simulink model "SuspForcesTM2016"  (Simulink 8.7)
settings: Solver=VariableStepAuto  SolverMode=SingleTasking  StartTime=0.0  StopTime=10.0  RelTol=1e-3

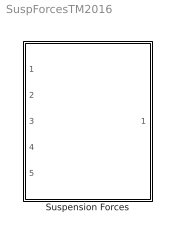
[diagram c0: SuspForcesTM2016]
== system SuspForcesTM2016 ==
  Suspension Forces : Subsystem

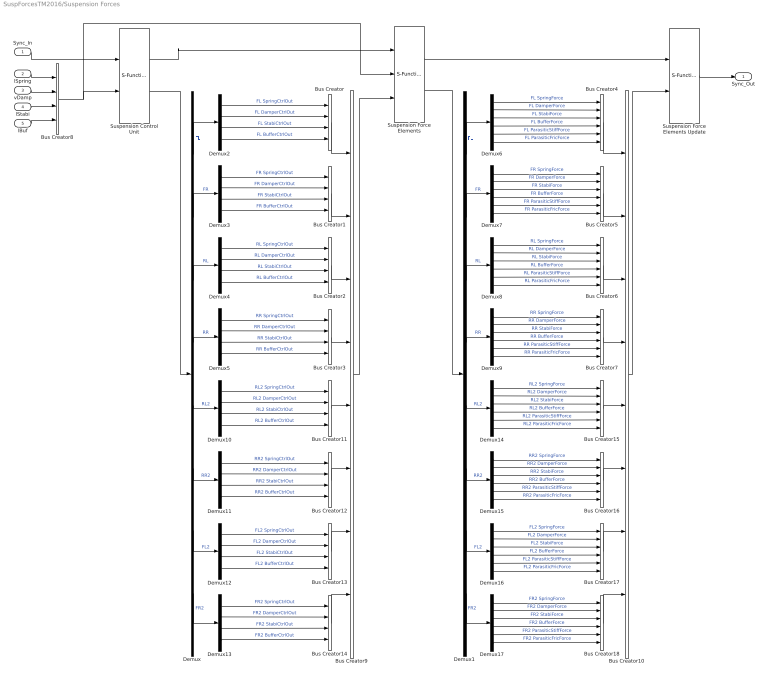
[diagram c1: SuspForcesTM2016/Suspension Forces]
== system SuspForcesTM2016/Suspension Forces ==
  Sync_In : Inport
  lSpring : Inport  Port=2
  vDamp : Inport  Port=3
  lStabi : Inport  Port=4
  lBuf : Inport  Port=5
  Bus Creator{,1..3,8,11..14} (9 alike) : BusCreator  Inputs=4
  Bus Creator10 : BusCreator  Inputs=8
  Bus Creator{4..7,15..18} (8 alike) : BusCreator  Inputs=6
  Bus Creator9 : BusCreator  Inputs=8
  Demux : Demux  Outputs=8
  Demux1 : Demux  Outputs=8
  Demux{2..5,10..13} (8 alike) : Demux
  Demux{6..9,14..17} (8 alike) : Demux  Outputs=6
  Suspension Control Unit : S-Function  FunctionName=TM_Sfun  Parameters='ForcesSuspControl'  SFunctionDeploymentMode=off  EnableBusSupport=off
  Suspension Force Elements : S-Function  FunctionName=TM_Sfun  Parameters='ForcesSusp'  SFunctionDeploymentMode=off  EnableBusSupport=off
  Suspension Force Elements Update : S-Function  FunctionName=TM_Sfun  Parameters='ForcesSuspUpd'  SFunctionDeploymentMode=off  EnableBusSupport=off
  Sync_Out : Outport
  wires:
  vDamp/1 -> Bus Creator8/2
  lStabi/1 -> Bus Creator8/3
  lBuf/1 -> Bus Creator8/4
  lSpring/1 -> Bus Creator8/1
  Bus Creator8/1 -> Suspension Control Unit/2, Suspension Force Elements/2
  Sync_In/1 -> Suspension Control Unit/1
  Suspension Control Unit/1 -> Suspension Force Elements/1
  Suspension Force Elements/1 -> Suspension Force Elements Update/1
  Suspension Force Elements Update/1 -> Sync_Out/1
  Bus Creator4/1 -> Bus Creator10/1
  Bus Creator5/1 -> Bus Creator10/2
  Bus Creator6/1 -> Bus Creator10/3
  Bus Creator7/1 -> Bus Creator10/4
  Demux6/1 -> Bus Creator4/1  "FL SpringForce"
  Demux9/1 -> Bus Creator7/1  "RR SpringForce"
  Demux9/2 -> Bus Creator7/2  "RR DamperForce"
  Demux9/3 -> Bus Creator7/3  "RR StabiForce"
  Demux9/4 -> Bus Creator7/4  "RR BufferForce"
  Demux9/5 -> Bus Creator7/5  "RR ParasiticStiffForce"
  Demux9/6 -> Bus Creator7/6  "RR ParasiticFricForce"
  Demux8/1 -> Bus Creator6/1  "RL SpringForce"
  Demux8/2 -> Bus Creator6/2  "RL DamperForce"
  Demux8/4 -> Bus Creator6/4  "RL BufferForce"
  Demux8/5 -> Bus Creator6/5  "RL ParasiticStiffForce"
  Demux8/6 -> Bus Creator6/6  "RL ParasiticFricForce"
  Demux8/3 -> Bus Creator6/3  "RL StabiForce"
  Demux7/1 -> Bus Creator5/1  "FR SpringForce"
  Demux7/2 -> Bus Creator5/2  "FR DamperForce"
  Demux7/3 -> Bus Creator5/3  "FR StabiForce"
  Demux7/4 -> Bus Creator5/4  "FR BufferForce"
  Demux7/5 -> Bus Creator5/5  "FR ParasiticStiffForce"
  Demux7/6 -> Bus Creator5/6  "FR ParasiticFricForce"
  Demux6/2 -> Bus Creator4/2  "FL DamperForce"
  Demux6/3 -> Bus Creator4/3  "FL StabiForce"
  Demux6/4 -> Bus Creator4/4  "FL BufferForce"
  Demux6/5 -> Bus Creator4/5  "FL ParasiticStiffForce"
  Demux6/6 -> Bus Creator4/6  "FL ParasiticFricForce"
  Bus Creator10/1 -> Suspension Force Elements Update/2
  Demux/1 -> Demux2/1  "FL"
  Bus Creator1/1 -> Bus Creator9/2
  Demux/2 -> Demux3/1  "FR"
  Bus Creator2/1 -> Bus Creator9/3
  Demux/3 -> Demux4/1  "RL"
  Bus Creator3/1 -> Bus Creator9/4
  Demux2/1 -> Bus Creator/1  "FL SpringCtrlOut"
  Demux/4 -> Demux5/1  "RR"
  Demux5/1 -> Bus Creator3/1  "RR SpringCtrlOut"
  Demux5/2 -> Bus Creator3/2  "RR DamperCtrlOut"
  Demux5/3 -> Bus Creator3/3  "RR StabiCtrlOut"
  Demux5/4 -> Bus Creator3/4  "RR BufferCtrlOut"
  Demux4/1 -> Bus Creator2/1  "RL SpringCtrlOut"
  Demux4/2 -> Bus Creator2/2  "RL DamperCtrlOut"
  Demux4/4 -> Bus Creator2/4  "RL BufferCtrlOut"
  Demux4/3 -> Bus Creator2/3  "RL StabiCtrlOut"
  Demux3/1 -> Bus Creator1/1  "FR SpringCtrlOut"
  Demux3/2 -> Bus Creator1/2  "FR DamperCtrlOut"
  Demux3/3 -> Bus Creator1/3  "FR StabiCtrlOut"
  Demux3/4 -> Bus Creator1/4  "FR BufferCtrlOut"
  Demux2/2 -> Bus Creator/2  "FL DamperCtrlOut"
  Demux2/3 -> Bus Creator/3  "FL StabiCtrlOut"
  Demux2/4 -> Bus Creator/4  "FL BufferCtrlOut"
  Suspension Control Unit/2 -> Demux/1
  Bus Creator9/1 -> Suspension Force Elements/3
  Bus Creator/1 -> Bus Creator9/1
  Suspension Force Elements/2 -> Demux1/1
  Demux1/1 -> Demux6/1  "FL"
  Demux1/2 -> Demux7/1  "FR"
  Demux1/3 -> Demux8/1  "RL"
  Demux1/4 -> Demux9/1  "RR"
  Demux/5 -> Demux10/1  "RL2"
  Bus Creator12/1 -> Bus Creator9/6
  Demux/6 -> Demux11/1  "RR2"
  Bus Creator13/1 -> Bus Creator9/7
  Demux/7 -> Demux12/1  "FL2"
  Bus Creator14/1 -> Bus Creator9/8
  Demux10/1 -> Bus Creator11/1  "RL2 SpringCtrlOut"
  Demux/8 -> Demux13/1  "FR2"
  Demux13/1 -> Bus Creator14/1  "FR2 SpringCtrlOut"
  Demux13/2 -> Bus Creator14/2  "FR2 DamperCtrlOut"
  Demux13/3 -> Bus Creator14/3  "FR2 StabiCtrlOut"
  Demux13/4 -> Bus Creator14/4  "FR2 BufferCtrlOut"
  Demux12/1 -> Bus Creator13/1  "FL2 SpringCtrlOut"
  Demux12/2 -> Bus Creator13/2  "FL2 DamperCtrlOut"
  Demux12/4 -> Bus Creator13/4  "FL2 BufferCtrlOut"
  Demux12/3 -> Bus Creator13/3  "FL2 StabiCtrlOut"
  Demux11/1 -> Bus Creator12/1  "RR2 SpringCtrlOut"
  Demux11/2 -> Bus Creator12/2  "RR2 DamperCtrlOut"
  Demux11/3 -> Bus Creator12/3  "RR2 StabiCtrlOut"
  Demux11/4 -> Bus Creator12/4  "RR2 BufferCtrlOut"
  Demux10/2 -> Bus Creator11/2  "RL2 DamperCtrlOut"
  Demux10/3 -> Bus Creator11/3  "RL2 StabiCtrlOut"
  Demux10/4 -> Bus Creator11/4  "RL2 BufferCtrlOut"
  Bus Creator11/1 -> Bus Creator9/5
  Bus Creator15/1 -> Bus Creator10/5
  Bus Creator16/1 -> Bus Creator10/6
  Bus Creator17/1 -> Bus Creator10/7
  Bus Creator18/1 -> Bus Creator10/8
  Demux14/1 -> Bus Creator15/1  "RL2 SpringForce"
  Demux17/1 -> Bus Creator18/1  "FR2 SpringForce"
  Demux17/2 -> Bus Creator18/2  "FR2 DamperForce"
  Demux17/3 -> Bus Creator18/3  "FR2 StabiForce"
  Demux17/4 -> Bus Creator18/4  "FR2 BufferForce"
  Demux17/5 -> Bus Creator18/5  "FR2 ParasiticStiffForce"
  Demux17/6 -> Bus Creator18/6  "FR2 ParasiticFricForce"
  Demux16/1 -> Bus Creator17/1  "FL2 SpringForce"
  Demux16/2 -> Bus Creator17/2  "FL2 DamperForce"
  Demux16/4 -> Bus Creator17/4  "FL2 BufferForce"
  Demux16/5 -> Bus Creator17/5  "FL2 ParasiticStiffForce"
  Demux16/6 -> Bus Creator17/6  "FL2 ParasiticFricForce"
  Demux16/3 -> Bus Creator17/3  "FL2 StabiForce"
  Demux15/1 -> Bus Creator16/1  "RR2 SpringForce"
  Demux15/2 -> Bus Creator16/2  "RR2 DamperForce"
  Demux15/3 -> Bus Creator16/3  "RR2 StabiForce"
  Demux15/4 -> Bus Creator16/4  "RR2 BufferForce"
  Demux15/5 -> Bus Creator16/5  "RR2 ParasiticStiffForce"
  Demux15/6 -> Bus Creator16/6  "RR2 ParasiticFricForce"
  Demux14/2 -> Bus Creator15/2  "RL2 DamperForce"
  Demux14/3 -> Bus Creator15/3  "RL2 StabiForce"
  Demux14/4 -> Bus Creator15/4  "RL2 BufferForce"
  Demux14/5 -> Bus Creator15/5  "RL2 ParasiticStiffForce"
  Demux14/6 -> Bus Creator15/6  "RL2 ParasiticFricForce"
  Demux1/5 -> Demux14/1  "RL2"
  Demux1/6 -> Demux15/1  "RR2"
  Demux1/7 -> Demux16/1  "FL2"
  Demux1/8 -> Demux17/1  "FR2"
